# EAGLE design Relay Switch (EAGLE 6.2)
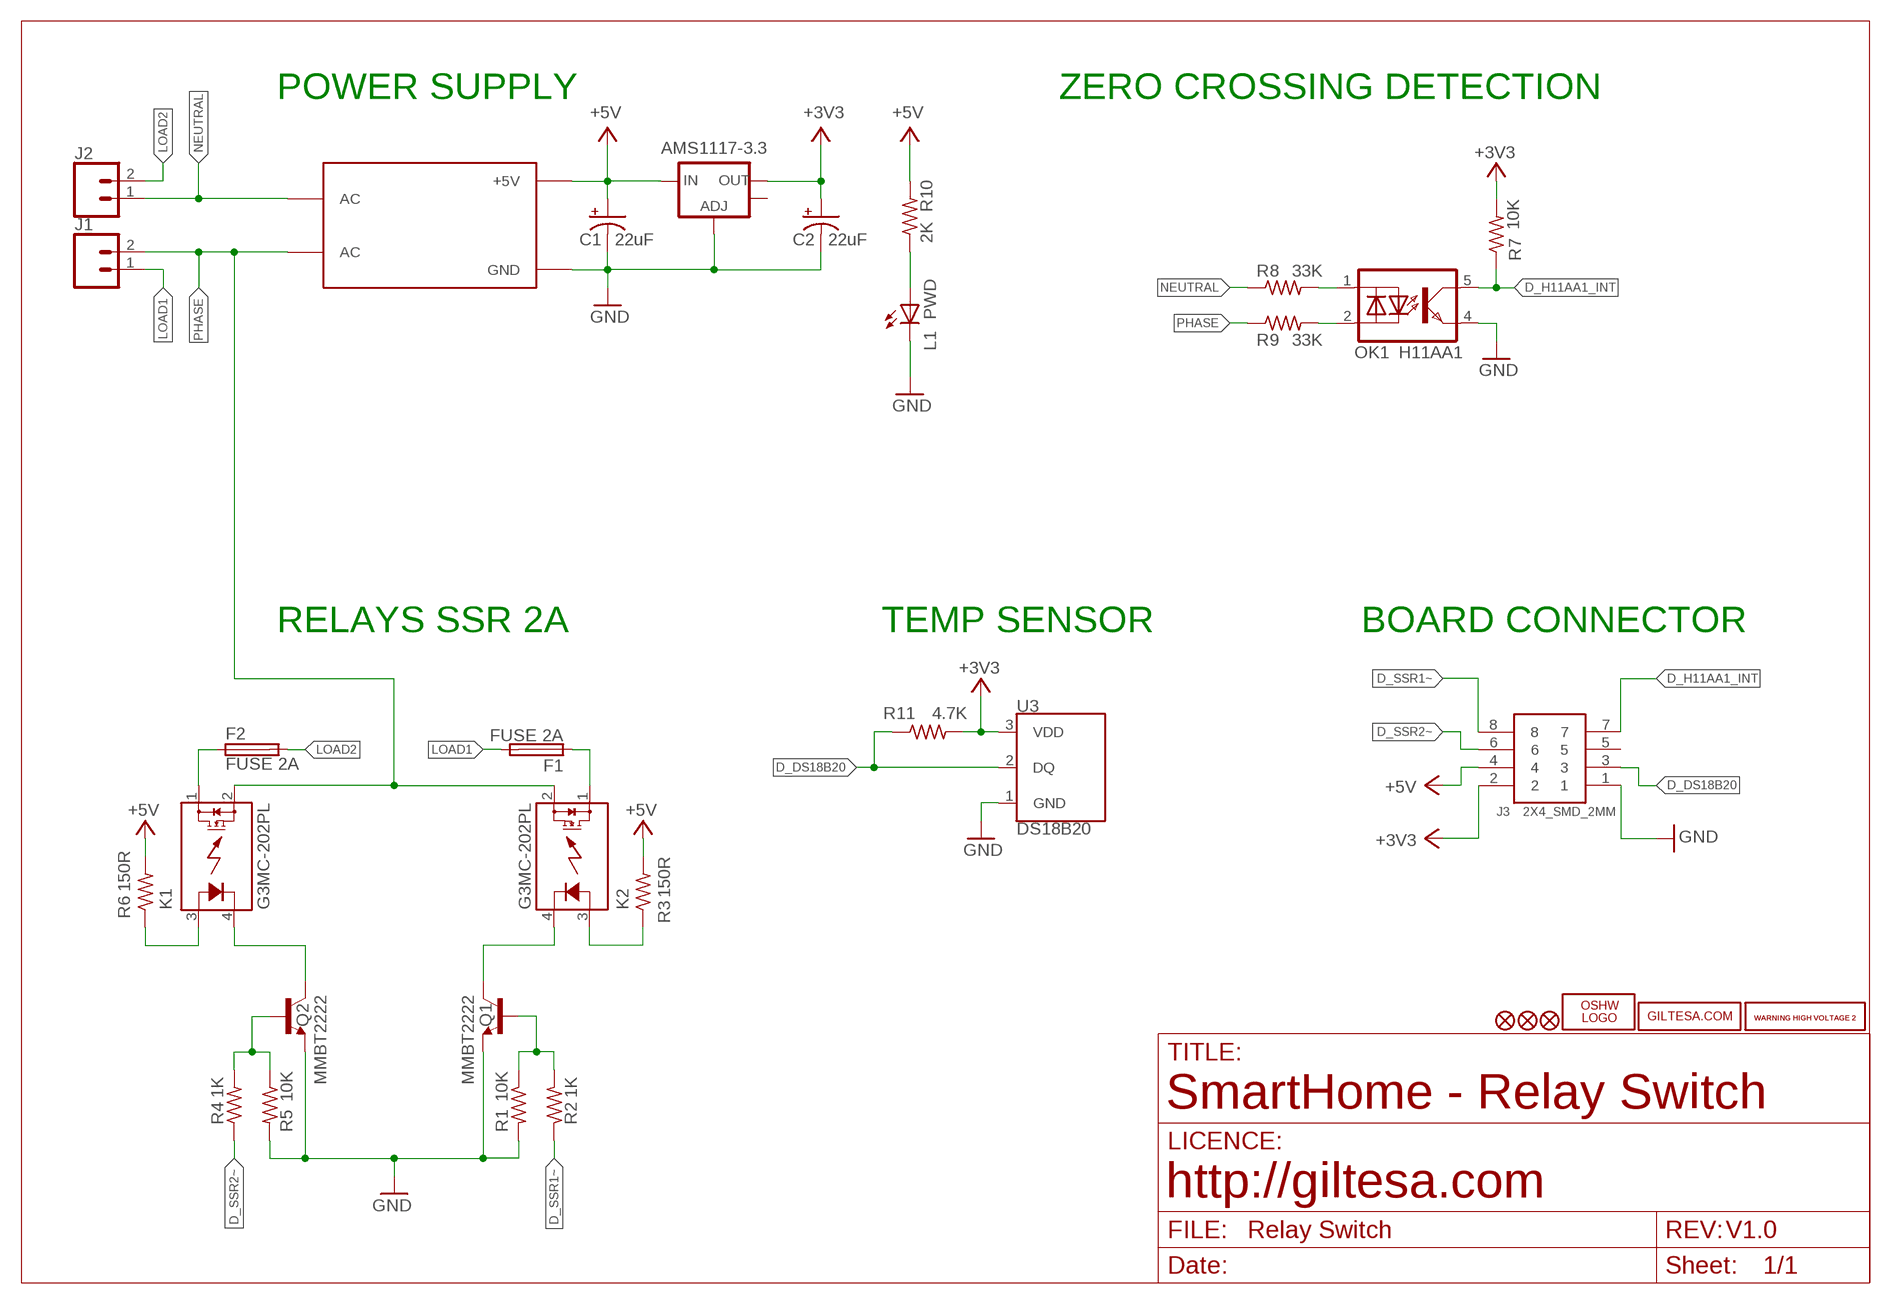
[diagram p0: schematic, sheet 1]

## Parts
AMS1117-3.3  V_REG_LM1117SOT223  [SOT223]
C1  22uF  CAP_POL3528  [EIA3528]
C2  22uF  CAP_POL3528  [EIA3528]
F1  FUSE 2A  FUSETE5  [TE5]
F2  FUSE 2A  FUSETE5  [TE5]
J1  TERMINAL_5MM_2P  [TERMINAL_5MM_2P]
J2  TERMINAL_5MM_2P  [TERMINAL_5MM_2P]
J3  2X4_SMD_2MM  2X4_SMD_2.0MM  [2X4_SMD_2.0MM]
K1  G3MC-202PL  RELAY_SSD_SPST  [RELAY_G3MB_SPST]
K2  G3MC-202PL  RELAY_SSD_SPST  [RELAY_G3MB_SPST]
L1  PWD  LEDCHIP-LED0805  [CHIP-LED0805]
LOGO1  OSHW_LOGO_FILLX0150-NT  [OSHW_FILLX150_NOTEXT]
OK1  H11AA1  [H11AA1]
Q1  MMBT2222  TRANSISTOR_NPNSOT23  [SOT23]
Q2  MMBT2222  TRANSISTOR_NPNSOT23  [SOT23]
R1  10K  R0603  [R0603]
R2  1K  R0603  [R0603]
R3  150R  R0603  [R0603]
R4  1K  R0603  [R0603]
R5  10K  R0603  [R0603]
R6  150R  R0603  [R0603]
R7  10K  R0603  [R0603]
R8  33K  R2010  [R2010]
R9  33K  R2010  [R2010]
R10  2K  R0603  [R0603]
R11  4.7K  R0603  [R0603]
U3  DS18B20  [DS18B20]
U$1  HILINK_HLK-PM01_5V  [HILINK_HLK-PM01_5V]
U$3  WARNING_HIGH_VOLTAGE_2  [WARNING_HIGH_VOLTAGE_2]
U$4  WARNING_HIGH_VOLTAGE_2  [WARNING_HIGH_VOLTAGE_2]
U$5  GILTESA.COM_MASK  [GILTESA.COM_MASK]
U$6  FIDUCIAL1X2  [FIDUCIAL-1X2]
U$7  FIDUCIAL1X2  [FIDUCIAL-1X2]
U$14  FIDUCIAL1X2  [FIDUCIAL-1X2]

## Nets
+3V3: AMS1117-3.3.2(OUT) C2.A(+) J3.2 R7.2 R11.2 U3.3(VDD)
+5V: AMS1117-3.3.3(IN) C1.A(+) J3.4 R3.2 R6.2 R10.2 U$1.+5V
D_DS18B20: J3.3 R11.1 U3.2(DQ)
D_H11AA1_INT: J3.7 OK1.5 R7.1
D_SSR1~: J3.8 R2.1
D_SSR2~: J3.6 R4.1
GND: AMS1117-3.3.1(ADJ) C1.C(-) C2.C(-) J3.1 L1.C OK1.4 Q1.2(E) Q2.2(E) R1.2 R5.2 U3.1(GND) U$1.GND
LOAD1: F1.2 J1.1
LOAD2: F2.2 J2.2
N$1: F1.1 K2.1
N$2: Q1.1(B) R1.1 R2.2
N$3: K2.4 Q1.3(C)
N$4: K2.3 R3.1
N$5: K1.3 R6.1
N$6: OK1.1 R8.2
N$7: OK1.2 R9.2
N$8: L1.A R10.1
N$9: F2.1 K1.1
N$46: Q2.1(B) R4.2 R5.1
N$47: K1.4 Q2.3(C)
NEUTRAL: J2.1 R8.1 U$1.AC@2(AC)
PHASE: J1.2 K1.2 K2.2 R9.1 U$1.AC@1(AC)
Unconnected: AMS1117-3.3.4(OUT) J3.5

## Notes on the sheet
- POWER SUPPLY | ZERO CROSSING DETECTION
- RELAYS SSR 2A | TEMP SENSOR | BOARD CONNECTOR
- SmartHome - Relay Switch
- http://giltesa.com
- V1.0

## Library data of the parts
AMS1117-3.3 = SparkFun:V_REG_LM1117: Voltage Regulator LM1117 Standard adjustable voltage regulator but in SMD form. Spark Fun Electronics SKU : COM-00595
C1 C2 = SparkFun:CAP_POL: Capacitor Polarized
F1 F2 = fuse:FUSE: Fuse; OC_FARNELL: unknown; OC_NEWARK: unknown
J1 J2 = ,giltesa:TERMINAL_5MM_2P
J3 = ,giltesa:2X4_SMD_2.0MM
K1 K2 = TD-MySensors:RELAY_SSD_SPST
L1 = led:LED: LED
LOGO1 = ohw-logo:OSHW_LOGO_FILL
OK1 = ,giltesa:H11AA1
Q1 Q2 = SparkFun:TRANSISTOR_NPN: Transistor NPN BJT configuration in SOT23 package. MMBT2222 is the common NPN we use. Double check BCE configuration again layout.
R1-R7 R10 R11 = ,giltesa:R0603
R8 R9 = ,giltesa:R2010
U3 = ,giltesa:DS18B20
U$1 = ,giltesa:HILINK_HLK-PM01_5V
U$3 U$4 = ,giltesa_logos:WARNING_HIGH_VOLTAGE_2
U$5 = ,giltesa_logos:GILTESA.COM_MASK
U$6 U$7 U$14 = SparkFun:FIDUCIAL: Fiducial Alignment Points

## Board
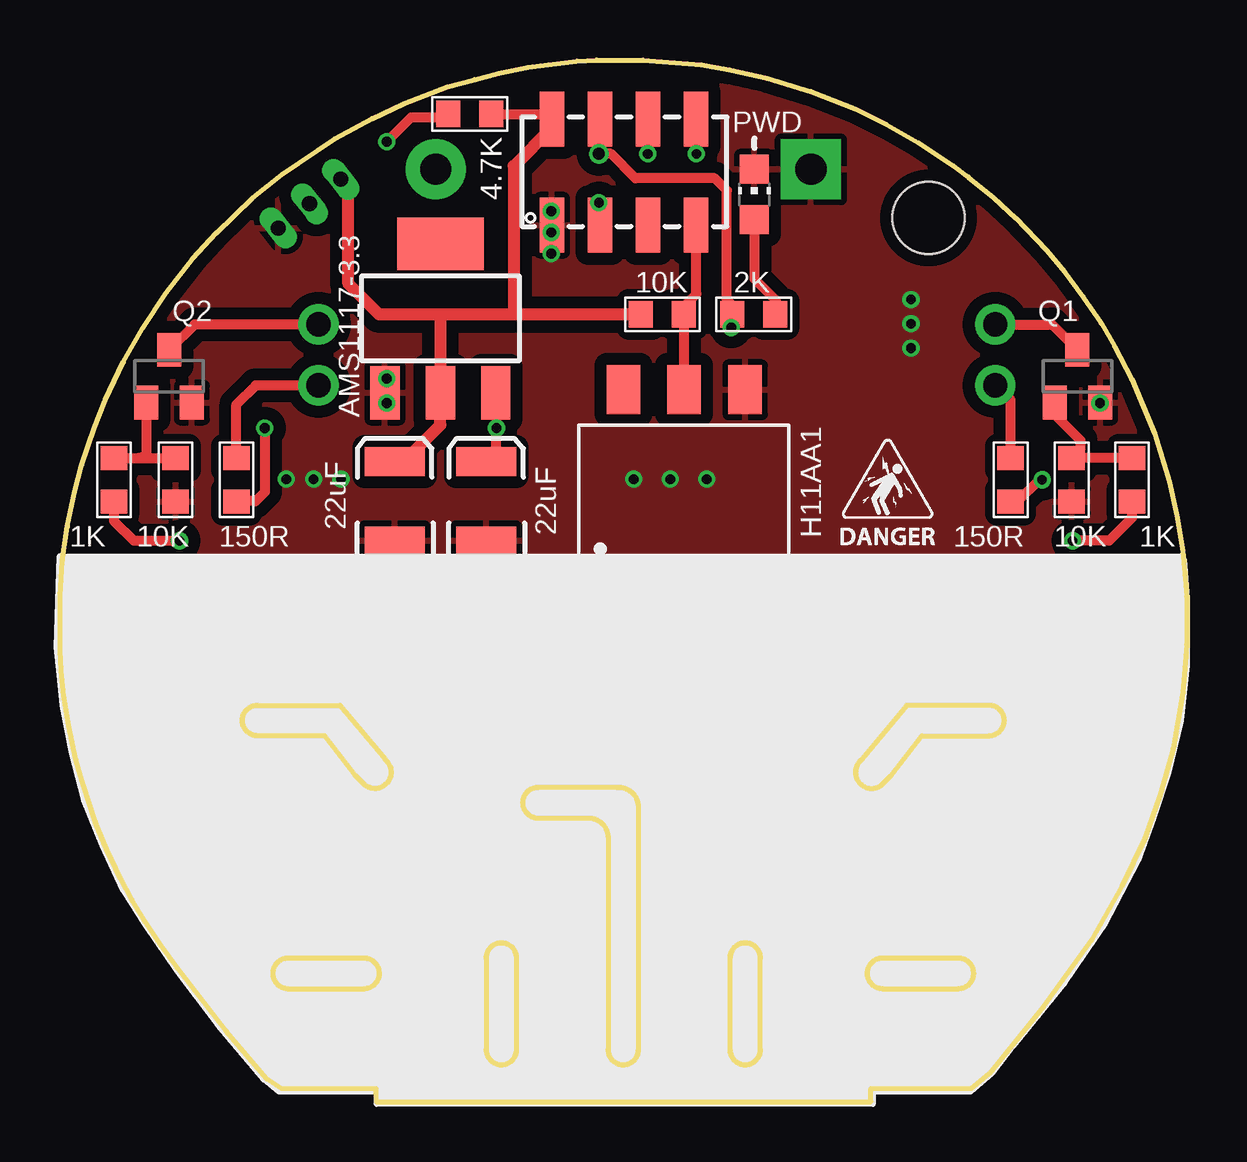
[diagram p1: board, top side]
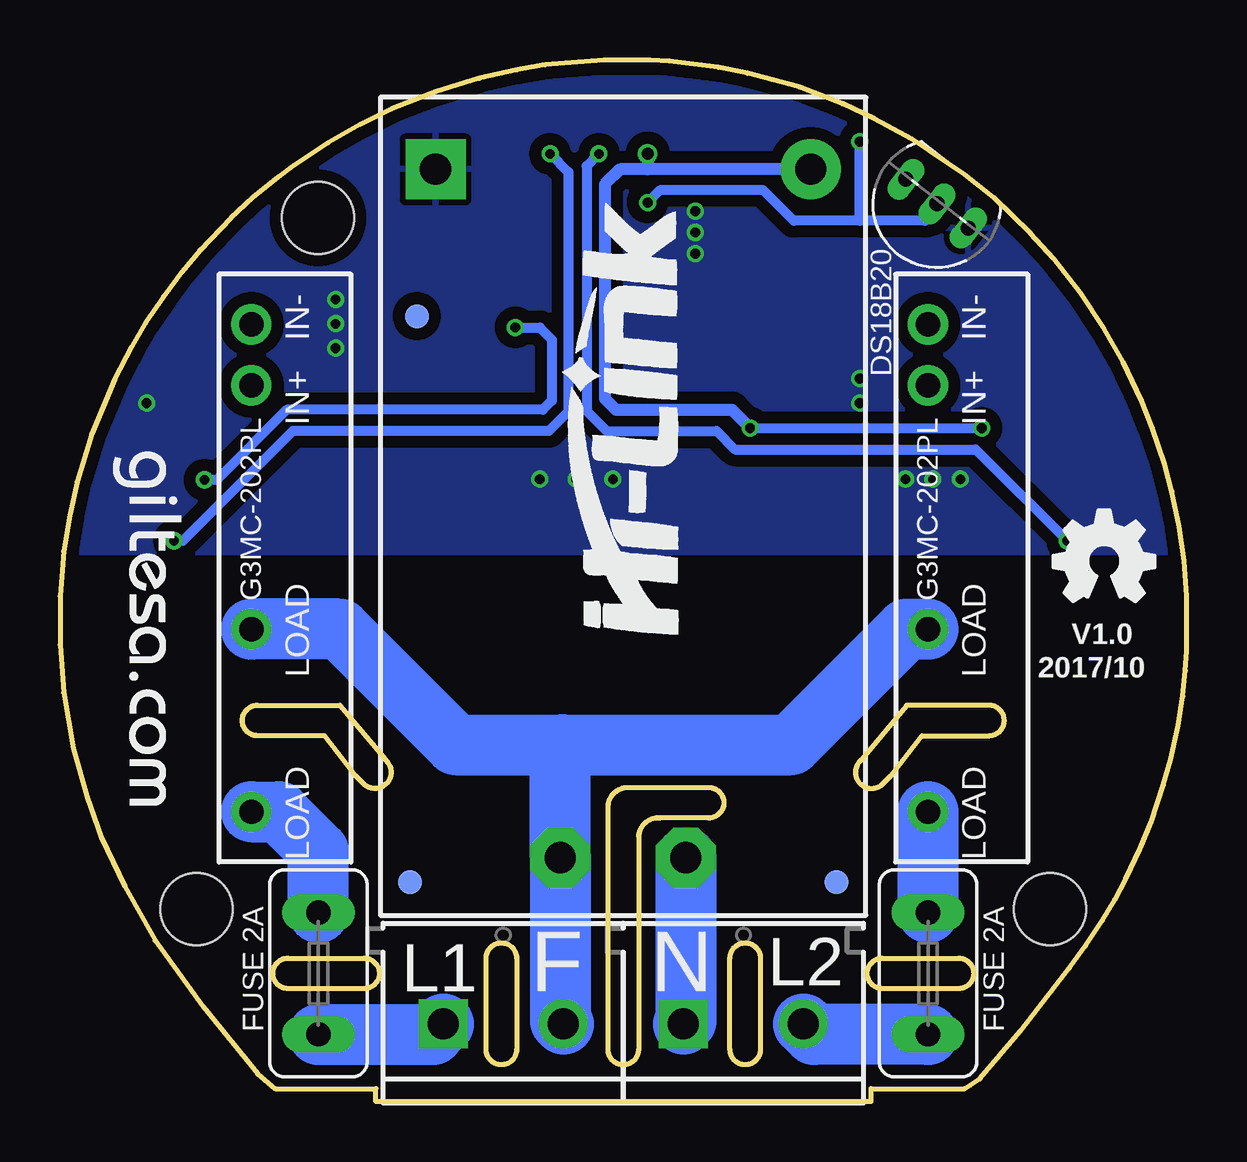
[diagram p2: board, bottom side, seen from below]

Size 46.94 x 43.43 mm. Coordinates in mm from the lower left corner, seen from the top.
Outline: 115 segments
Copper layers (1*16): Top 0.035mm / dielectric 1.6mm / Bottom 0.035mm
Design rules: minimum track width 6mil, minimum drill 12mil, track to track 6mil, track to pad 6mil, pad to pad 6mil, via to via 8mil, smd to smd 0mil, copper to edge 20mil, drill to drill 10mil, minimum pad ring 6mil, minimum via ring 6mil, stop-mask expansion 0mil, vias tented up to drill 100mil, thermal gap 10mil
Holes 3 mm at 5.69,8.03 41.25,8.03 36.19,36.84

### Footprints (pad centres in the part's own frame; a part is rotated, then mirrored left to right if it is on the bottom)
SOT223 = smd 1.219 x 2.235: 1 -2.311,-3.099; 2 0,-3.099; 3 2.311,-3.099 | smd 3.6 x 2.2: 4 0,3.099
EIA3528 = smd 1.2 x 2.5: A 1.65,0; C -1.65,0
TE5 = drill 1.016 long: 1 -2.54,0; 2 2.54,0
TERMINAL_5MM_2P = drill 1.3 pad 2.032 square: 1 0,0 | drill 1.3 pad 2.032: 2 5,0
2X4_SMD_2.0MM = smd 2.286 x 1.016: 1 -2.213,2.976; 2 2.212,2.976; 3 -2.213,0.976; 4 2.212,0.976; 5 -2.213,-1.024; 6 2.212,-1.024; 7 -2.213,-3.024; 8 2.212,-3.024
RELAY_G3MB_SPST = drill 1.016 pad 1.676: 1 10.16,-1.4; 2 2.54,-1.4; 3 -7.62,-1.4; 4 -10.16,-1.4
CHIP-LED0805 = smd 1.2 x 1.2: A 0,-1.05; C 0,1.05
H11AA1 = smd 1.397 x 2.032: 1 -2.54,-4.645; 2 0,-4.645; 3 2.54,-4.645; 4 2.54,4.645; 5 0,4.645; 6 -2.54,4.645
SOT23 = smd 1 x 1.4: 1 -0.95,-1.1; 2 0.95,-1.1; 3 0,1.1
R0603 = smd 1 x 1.1: 1 -0.901,0.013; 2 0.901,0.013
R2010 = smd 1.8 x 2.7: 1 -2.2,0; 2 2.2,0
DS18B20 = drill 0.635 pad 0.864 long: 1 -1.651,0; 2 0,0; 3 1.651,0
HILINK_HLK-PM01_5V = drill 1.3 pad 2.5: +5V 31.109,2.3 | drill 1.3 pad 2.5 octagon: AC@1 2.409,12.73; AC@2 2.409,7.5 | drill 1.3 pad 2.5 square: GND 31.109,17.93
FIDUCIAL-1X2 = smd 1 x 1: 1 0,0

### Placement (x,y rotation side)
AMS1117-3.3  15.85,32.66 0 top
C1  17.75,25.04 90 top
C2  13.94,25.04 90 top
F1  36.17,5.35 270 bottom
F2  10.77,5.35 270 bottom
J1  30.97,3.25 0 bottom
J2  20.97,3.25 0 bottom
J3  23.47,38.75 90 top
K1  9.37,22.24 270 bottom
K2  37.57,22.24 270 bottom
L1  28.93,37.83 0 top
LOGO1  5.56,20.85 0 bottom
OK1  26.01,25.04 0 top
Q1  42.39,30.24 0 top
Q2  4.55,30.24 0 top
R1  42.14,25.93 270 top
R2  44.68,25.93 90 top
R3  39.6,25.93 270 top
R4  2.26,25.93 90 top
R5  4.8,25.93 270 top
R6  7.34,25.93 270 top
R7  25.1,32.83 180 top
R8  17.5,14.62 90 top
R9  29.57,14.62 90 top
R10  28.91,32.83 180 top
R11  17.07,41.16 0 top
U3  10.4,37.44 142 bottom
U$1  13.36,7.76 90 bottom
U$2  [ELECTROCUTION_SMALL]  32.3,23.09 0 top
U$3  2.39,10.56 0 top
U$4  41,10.94 0 top
U$5  44.81,27.2 270 bottom
U$6  32.36,9.16 90 bottom
U$7  14.58,9.16 90 bottom
U$14  32.07,32.74 90 bottom

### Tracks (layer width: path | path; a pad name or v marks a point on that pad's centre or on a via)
+3V3
  Top 0.406: R11.2 20.49,41.17 J3.2
  Top 0.508: C2.A 14.2,26.56 15.85,28.21 AMS1117-3.3.2 15.85,32.82 | J3.2 20.49,40.6 18.9,39.01 18.9,32.82 | R7.2 18.9,32.82 | 18.9,32.82 15.85,32.82 | 15.85,32.82 13.3,32.82 12.02,34.1 12.02,37.93 U3.3
+5V  (via drill 0.41, 0.51)
  Top 0.406: v22.45,39.51 22.96,39.51 23.98,38.5 27.28,38.5 27.79,37.99 27.79,33.42 28,33.2 R10.2 28,32.31 v27.97,32.28 | v8.53,28.08 8.53,25.42 8.15,25.04 7.37,25.04 R6.2 | 18.19,26.81 v18.19,28.08 18.19,29.53 | 39.62,25.04 R3.2 39.89,25.02 40.79,25.93 v40.92,25.93
  Top 0.508: 18.14,29.53 AMS1117-3.3.3 18.19,29.53 | J3.4 22.49,39.81 v22.45,39.51 | C1.A 18.06,26.69 18.19,26.81
  Bottom 0.406: v18.19,28.08 v8.53,28.08 | v27.97,32.28 26.95,32.28 26.44,31.77 26.44,29.23 26.82,28.85 37.49,28.85 40.41,25.93 v40.92,25.93
  Bottom 0.508: U$1.+5V 22.45,38.87 | 22.45,38.87 23.6,38.87 24.23,38.24 24.23,29.3 23.77,28.85 18.95,28.85 v18.19,28.08 | v22.45,39.51 22.45,38.87
D_DS18B20  (via drill 0.41)
  Top 0.406: v22.45,37.48 22.45,36.58 J3.3 | v13.61,40.02 14.63,41.04 16.04,41.04 arc90 R11.1
  Bottom 0.406: U3.2 10.56,37.05 10.9,36.72 13.61,36.72 | 13.61,36.72 16.36,36.72 17.63,37.99 21.95,37.99 v22.45,37.48 | 13.61,36.72 v13.61,40.02
D_H11AA1_INT
  Top 0.406: OK1.5 26,29.7 R7.1 26,33.15 26.52,33.67 26.52,36.51 J3.7
D_SSR1~  (via drill 0.41)
  Top 0.406: v26.52,39.51 26.52,40.94 J3.8 | R2.1 44.67,24.34 43.71,23.39 v42.19,23.39
  Bottom 0.406: v26.52,39.51 25.76,38.75 25.76,28.77 26.57,27.96 37.24,27.96 41.81,23.39 v42.19,23.39
D_SSR2~  (via drill 0.41)
  Top 0.406: v24.49,39.51 J3.6 | R4.1 2.25,24.21 3.07,23.39 v4.98,23.39
  Bottom 0.406: v24.49,39.51 24.99,39.01 24.99,28.8 24.16,27.96 19.58,27.96 18.82,27.2 8.79,27.2 v4.98,23.39
GND  (via drill 0.41)
  other vias: 43.33,29.13 25.43,25.95 13.61,30.14 13.61,29.13 20.47,37.13 20.47,36.24 20.47,35.35 35.46,33.44 35.46,32.43 35.46,31.41 23.9,25.95 26.95,25.95 9.42,25.95 10.57,25.95 11.71,25.95
  pour Top (isolate 0.508): -0.03,22.88 46.96,22.88 46.96,23.77 46.33,26.31 45.06,29.48 42.52,33.93 39.98,37.1 35.53,40.28 29.82,42.82 24.74,43.45 20.93,43.45 15.85,42.18 10.77,39.64 6.96,36.47 3.78,32.66 1.88,29.48 -0.03,23.77
  pour Bottom (isolate 0.508): -0.03,22.88 46.96,22.88 46.33,26.31 45.06,29.48 42.52,33.93 39.98,37.1 35.53,40.28 29.82,42.82 24.74,43.45 20.93,43.45 15.85,42.18 10.77,39.64 6.96,36.47 3.78,32.66 1.88,29.48
LOAD1
  Bottom 2.54: F1.2 31.4,2.81 J1.1
LOAD2
  Bottom 2.54: F2.2 15.53,2.81 J2.2
N$1
  Bottom 2.54: F1.1 36.17,10.43 37.82,12.08 K2.1
N$2
  Top 0.406: R2.2 R1.1 42.52,27.22 42.52,27.58 41.44,28.65 Q1.1
N$3
  Top 0.406: K2.4 41.33,32.4 Q1.3
N$4
  Top 0.406: K2.3 39.01,29.86 39.61,29.27 R3.1
N$5
  Top 0.406: K1.3 8.15,29.86 7.35,29.06 R6.1
N$6
  Top 1.27: OK1.1 23.47,18.05 22.2,16.78 17.54,16.78 R8.2
N$7
  Top 1.27: OK1.2 26.01,18.05 27.28,16.78 29.52,16.78 R9.2
N$8
  Top 0.406: L1.A 28.93,34.31 29.82,33.42 29.82,32.84 R10.1
N$9
  Bottom 2.54: K1.1 F2.1
N$46
  Top 0.406: R4.2 3.28,26.83 | 3.28,26.83 R5.1 | Q2.1 3.6,26.89 3.28,26.83
N$47
  Top 0.406: K1.4 5.61,32.4 Q2.3
NEUTRAL
  Top 1.27: U$1.AC@2 19.28,10.17 17.75,11.7 17.75,12.17 R8.1
  Bottom 2.54: U$1.AC@2 20.86,3.35 J2.1
PHASE
  Top 1.27: R9.1 29.57,12.08 27.66,10.17 U$1.AC@1
  Bottom 2.54: 26.01,14.88 30.45,14.88 35.28,19.7 K2.2 | 26.01,14.88 16.48,14.88 11.66,19.7 K1.2 | 26.01,14.88 26.09,14.8 U$1.AC@1 26.09,3.37 J1.2

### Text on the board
bPlace: V1.0 | 2017/10 | L2 | N | F | L1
